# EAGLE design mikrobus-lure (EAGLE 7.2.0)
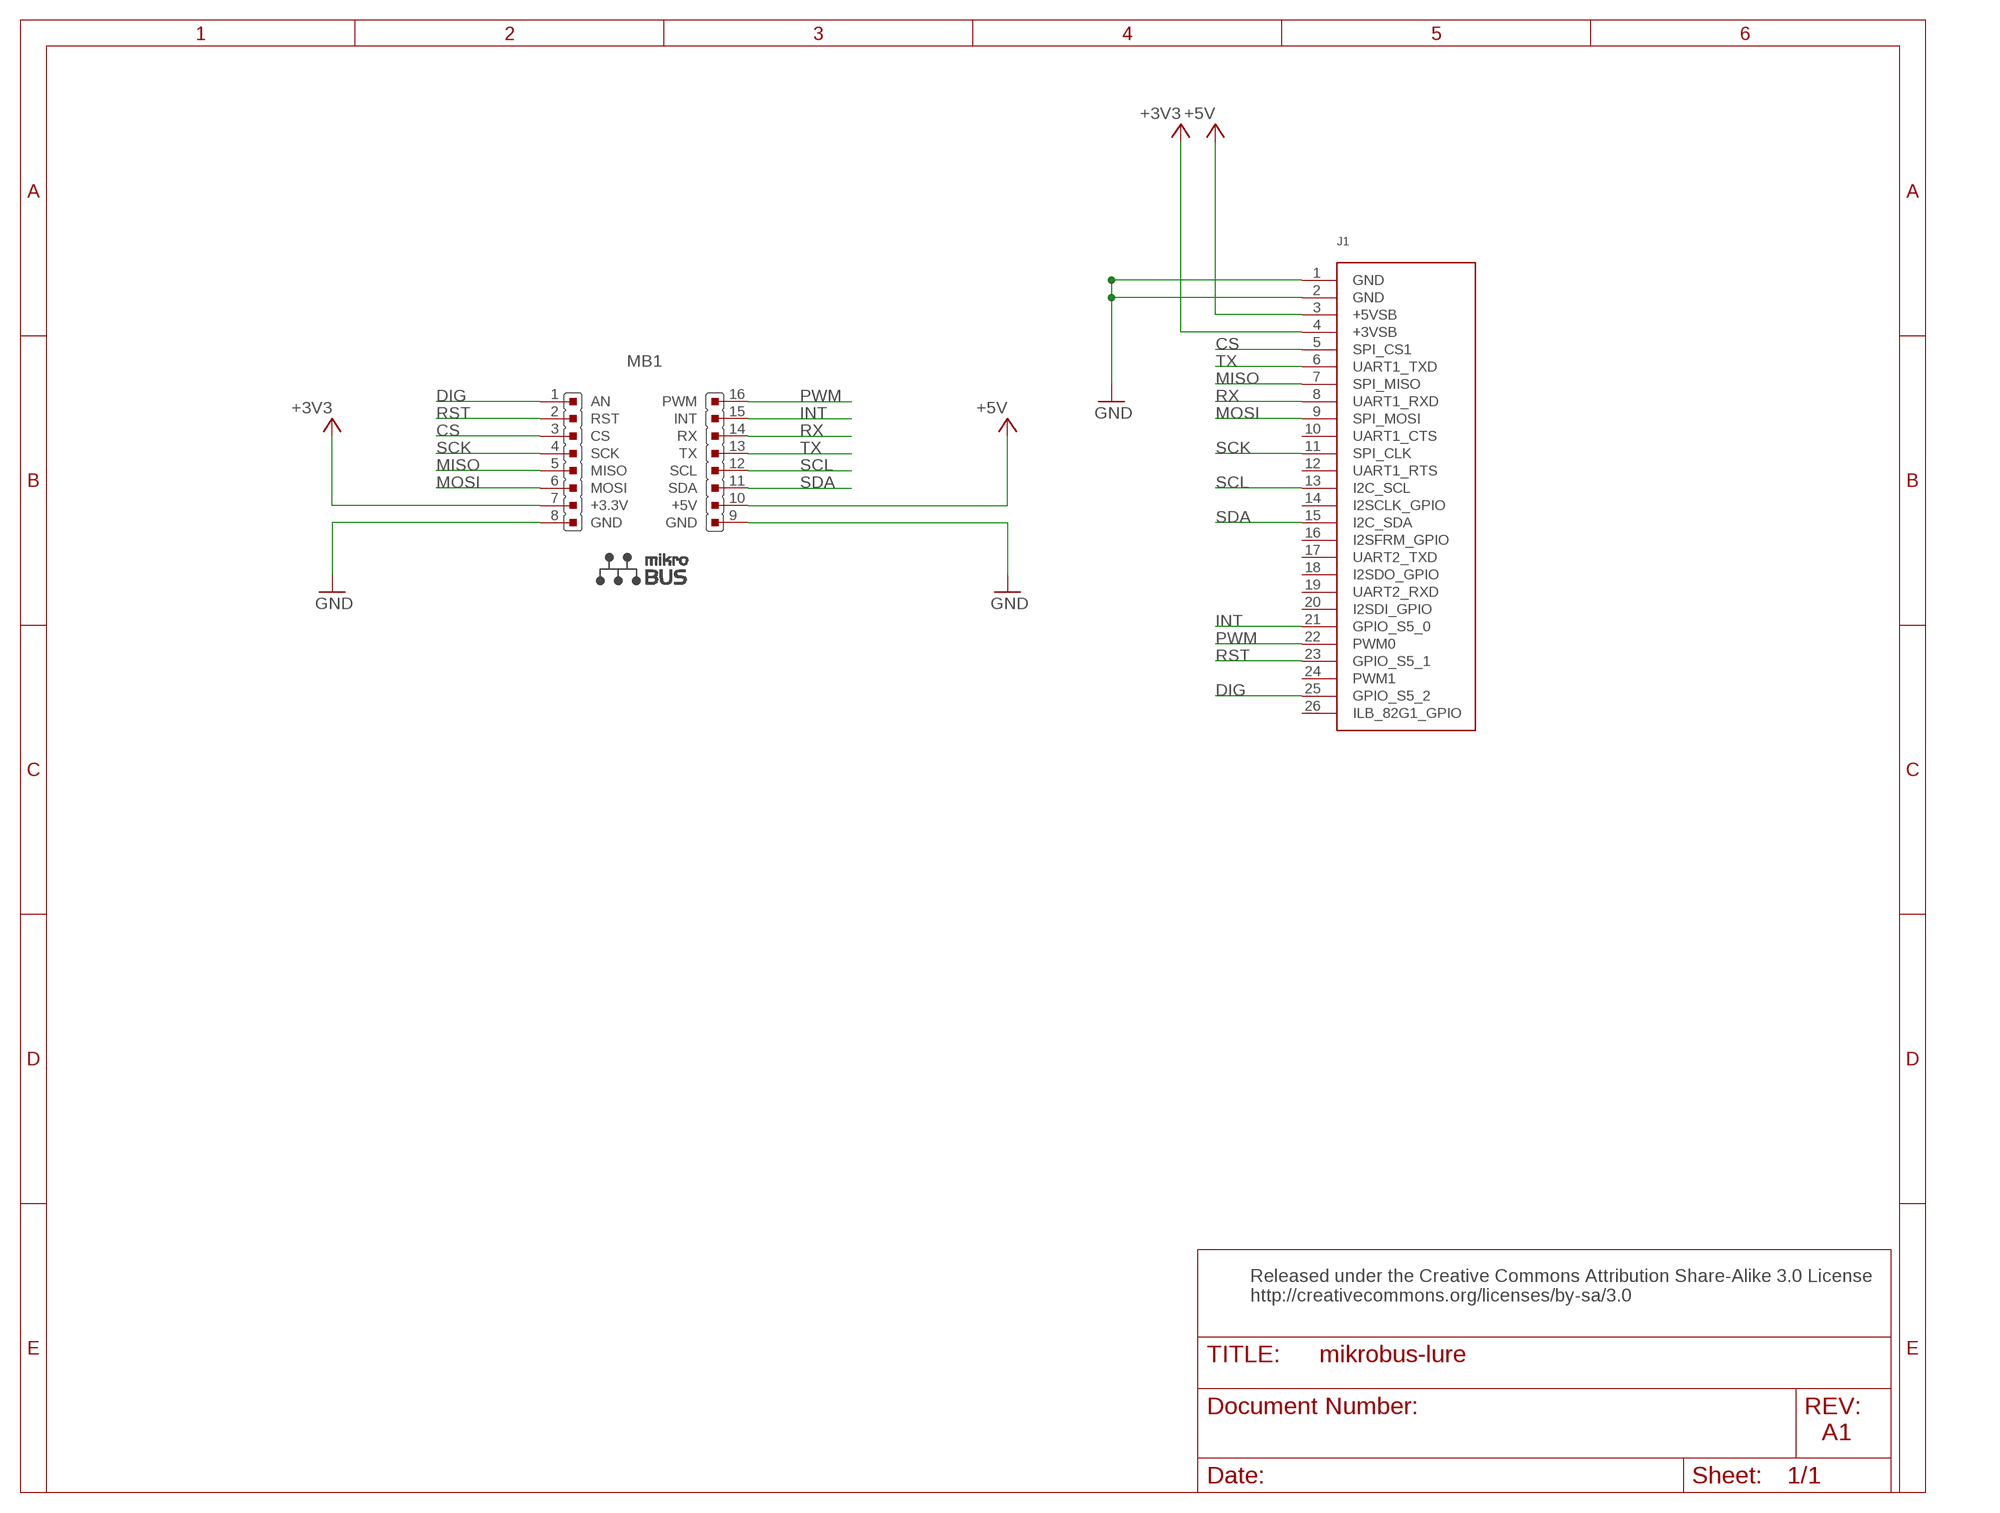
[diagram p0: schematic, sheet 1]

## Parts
J1  MBM_LSE  [MBM_LSE]
MB1  MIKROBUS  [MIKROBUS]

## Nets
+3V3: J1.4(+3VSB) MB1.7(+3.3V)
+5V: J1.3(+5VSB) MB1.10(+5V)
CS: J1.5(SPI_CS1) MB1.3(CS)
DIG: J1.25(GPIO_S5_2) MB1.1(AN)
GND: J1.1(GND) J1.2(GND) MB1.8(GND) MB1.9(GND)
INT: J1.21(GPIO_S5_0) MB1.15(INT)
MISO: J1.7(SPI_MISO) MB1.5(MISO)
MOSI: J1.9(SPI_MOSI) MB1.6(MOSI)
PWM: J1.22(PWM0) MB1.16(PWM)
RST: J1.23(GPIO_S5_1) MB1.2(RST)
RX: J1.8(UART1_RXD) MB1.14(RX)
SCK: J1.11(SPI_CLK) MB1.4(SCK)
SCL: J1.13(I2C_SCL) MB1.12(SCL)
SDA: J1.15(I2C_SDA) MB1.11(SDA)
TX: J1.6(UART1_TXD) MB1.13(TX)
Unconnected: J1.10(UART1_CTS) J1.12(UART1_RTS) J1.14(I2SCLK_GPIO) J1.16(I2SFRM_GPIO) J1.17(UART2_TXD) J1.18(I2SDO_GPIO) J1.19(UART2_RXD) J1.20(I2SDI_GPIO) J1.24(PWM1) J1.26(ILB_82G1_GPIO)

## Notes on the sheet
- Released under the Creative Commons Attribution Share-Alike 3.0 License
  http://creativecommons.org/licenses/by-sa/3.0
- A1

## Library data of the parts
J1 = mini-lse-lure:MBM_LSE
MB1 = MikroBUS:MIKROBUS: MikroBUS Source: MikroBUS specification MikroBUS

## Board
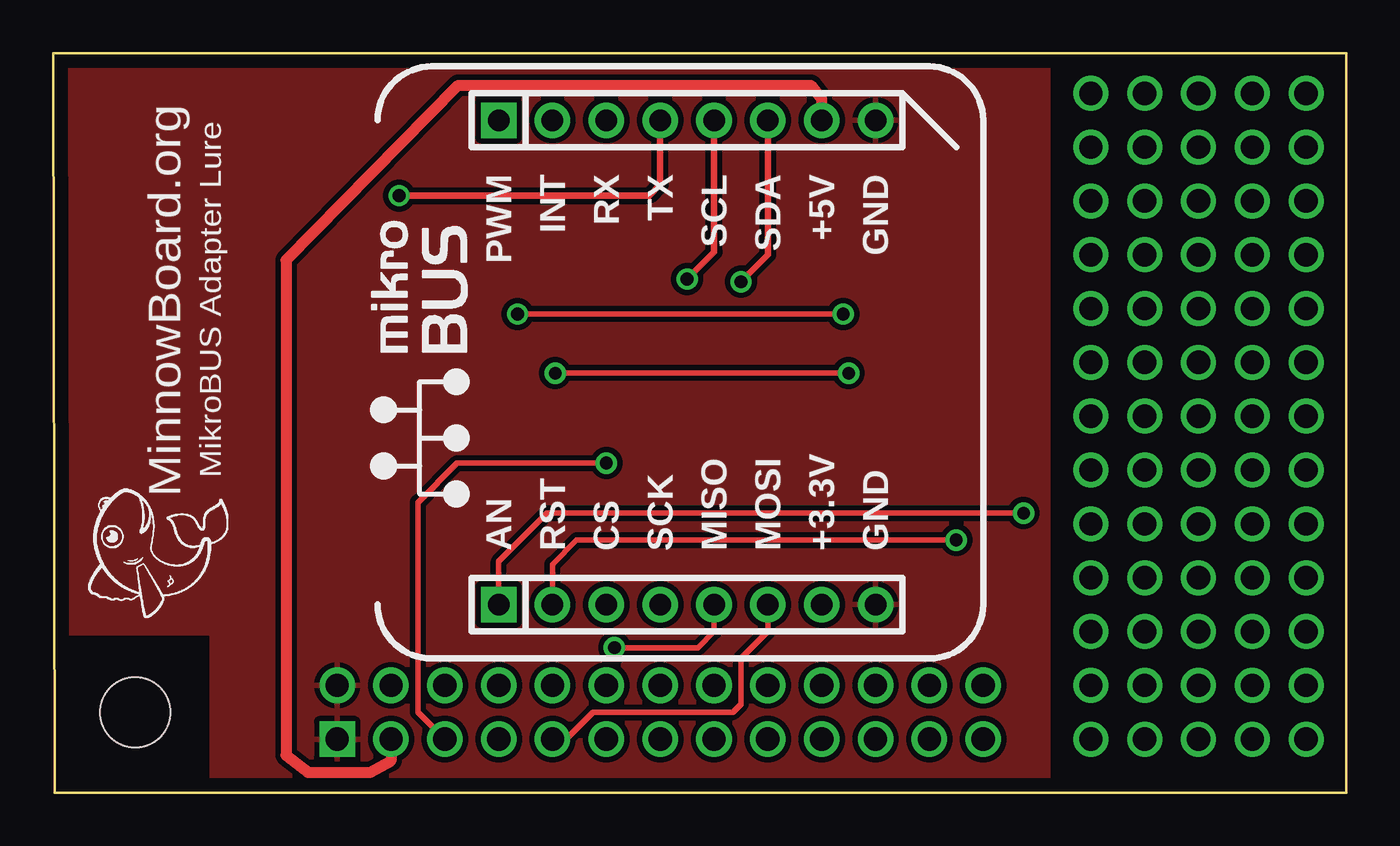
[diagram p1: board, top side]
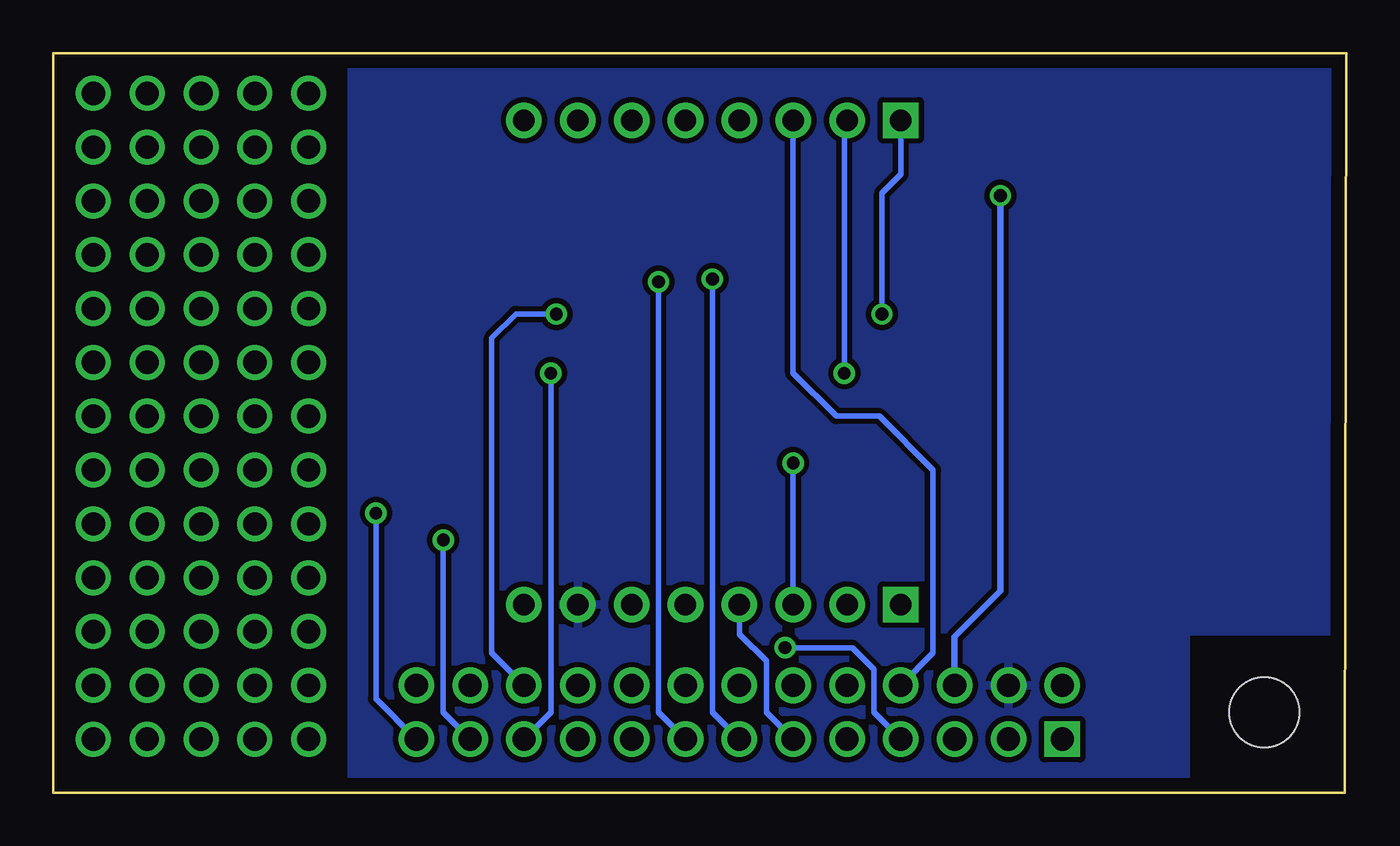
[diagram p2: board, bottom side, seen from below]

Size 61.04 x 34.92 mm. Coordinates in mm from the lower left corner, seen from the top.
Copper layers (1*16): Top 0.035mm / dielectric 1.5mm / Bottom 0.035mm
Design rules "default *": minimum track width 10mil, minimum drill 24mil, track to track 10mil, track to pad 10mil, pad to pad 10mil, via to via 10mil, smd to smd 8mil, copper to edge 25mil, drill to drill 8mil, minimum pad ring 0mil, minimum via ring 8mil, stop-mask expansion 4mil, vias tented up to drill 0mil, thermal gap 10mil

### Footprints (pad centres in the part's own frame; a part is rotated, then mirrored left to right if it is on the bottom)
MBM_LSE = drill 1.1 pad 1.676 square: 1 -15.24,0 | drill 1.1 pad 1.676: 2 -15.24,2.54; 3 -12.7,0; 4 -12.7,2.54; 5 -10.16,0; 6 -10.16,2.54; 7 -7.62,0; 8 -7.62,2.54; 9 -5.08,0; 10 -5.08,2.54; 11 -2.54,0; 12 -2.54,2.54; 13 0,0; 14 0,2.54; 15 2.54,0; 16 2.54,2.54; 17 5.08,0; 18 5.08,2.54; 19 7.62,0; 20 7.62,2.54; 21 10.16,0; 22 10.16,2.54; 23 12.7,0; 24 12.7,2.54; 25 15.24,0; 26 15.24,2.54 | hole 3.302: -24.765,1.27
MIKROBUS = drill 1.016 pad 1.676 square: 1 -11.43,7.62; 16 11.43,7.62 | drill 1.016 pad 1.676: 2 -11.43,5.08; 3 -11.43,2.54; 4 -11.43,0; 5 -11.43,-2.54; 6 -11.43,-5.08; 7 -11.43,-7.62; 8 -11.43,-10.16; 9 11.43,-10.16; 10 11.43,-7.62; 11 11.43,-5.08; 12 11.43,-2.54; 13 11.43,0; 14 11.43,2.54; 15 11.43,5.08

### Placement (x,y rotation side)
J1  28.65,2.54 0 top
MB1  28.65,20.32 90 top
U$1  [MINNOWBOARD_LOGO]  8.25,7.95 90 top

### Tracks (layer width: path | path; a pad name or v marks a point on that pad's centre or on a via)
+3V3
  pour Bottom: 0.08,34.92 46.94,34.92 46.94,0 0.08,0
+5V
  Top 0.508: J1.3 15.95,1.52 14.96,0.96 12.04,0.96 11,1.78 11,25.15 19.13,33.4 35.76,33.4 36.27,32.77 MB1.10
CS  (via drill 0.6)
  Top 0.254: J1.5 17.22,3.81 17.22,13.72 19.08,15.57 v26.11,15.57
  Bottom 0.254: v26.11,15.57 MB1.3
DIG  (via drill 0.6)
  Top 0.254: MB1.1 21.03,10.92 23.32,13.21 v45.8,13.21
  Bottom 0.254: v45.8,13.21 45.8,4.45 J1.25
GND
  pour Top: 0.08,34.92 46.94,34.92 46.94,0 0.08,0
INT  (via drill 0.6)
  Top 0.254: v37.54,19.81 v23.7,19.81
  Bottom 0.254: J1.21 37.54,3.81 v37.54,19.81 | v23.7,19.81 23.7,31.75 MB1.15
MISO  (via drill 0.6)
  Top 0.254: v26.49,6.86 30.43,6.86 31.19,7.62 MB1.5
  Bottom 0.254: J1.7 22.3,3.81 22.3,5.84 23.32,6.86 v26.49,6.86
MOSI
  Top 0.254: J1.9 24.21,2.54 25.48,3.81 32.08,3.81 32.46,4.19 32.46,6.35 33.73,7.62 MB1.6
N$16  (via drill 1.1)
  other vias: 59.13,2.54
N$17  (via drill 1.1)
  other vias: 59.13,5.08
N$18  (via drill 1.1)
  other vias: 59.13,7.62
N$19  (via drill 1.1)
  other vias: 59.13,10.16
N$20  (via drill 1.1)
  other vias: 59.13,12.7
N$21  (via drill 1.1)
  other vias: 59.13,15.24
N$22  (via drill 1.1)
  other vias: 59.13,17.78
N$23  (via drill 1.1)
  other vias: 59.13,20.32
N$24  (via drill 1.1)
  other vias: 59.13,22.86
N$25  (via drill 1.1)
  other vias: 59.13,25.4
N$26  (via drill 1.1)
  other vias: 59.13,27.94
N$27  (via drill 1.1)
  other vias: 59.13,30.48
N$28  (via drill 1.1)
  other vias: 59.13,33.02
N$31  (via drill 1.1)
  other vias: 56.59,2.54
N$32  (via drill 1.1)
  other vias: 56.59,5.08
N$33  (via drill 1.1)
  other vias: 56.59,7.62
N$34  (via drill 1.1)
  other vias: 56.59,10.16
N$35  (via drill 1.1)
  other vias: 56.59,12.7
N$36  (via drill 1.1)
  other vias: 56.59,15.24
N$37  (via drill 1.1)
  other vias: 56.59,17.78
N$38  (via drill 1.1)
  other vias: 56.59,20.32
N$39  (via drill 1.1)
  other vias: 56.59,22.86
N$40  (via drill 1.1)
  other vias: 56.59,25.4
N$41  (via drill 1.1)
  other vias: 56.59,27.94
N$42  (via drill 1.1)
  other vias: 56.59,30.48
N$43  (via drill 1.1)
  other vias: 56.59,33.02
N$46  (via drill 1.1)
  other vias: 54.05,2.54
N$47  (via drill 1.1)
  other vias: 54.05,5.08
N$48  (via drill 1.1)
  other vias: 54.05,7.62
N$49  (via drill 1.1)
  other vias: 54.05,10.16
N$50  (via drill 1.1)
  other vias: 54.05,12.7
N$51  (via drill 1.1)
  other vias: 54.05,15.24
N$52  (via drill 1.1)
  other vias: 54.05,17.78
N$53  (via drill 1.1)
  other vias: 54.05,20.32
N$54  (via drill 1.1)
  other vias: 54.05,22.86
N$55  (via drill 1.1)
  other vias: 54.05,25.4
N$56  (via drill 1.1)
  other vias: 54.05,27.94
N$57  (via drill 1.1)
  other vias: 54.05,30.48
N$58  (via drill 1.1)
  other vias: 54.05,33.02
N$61  (via drill 1.1)
  other vias: 51.51,2.54
N$62  (via drill 1.1)
  other vias: 51.51,5.08
N$63  (via drill 1.1)
  other vias: 51.51,7.62
N$64  (via drill 1.1)
  other vias: 51.51,10.16
N$65  (via drill 1.1)
  other vias: 51.51,12.7
N$66  (via drill 1.1)
  other vias: 51.51,15.24
N$67  (via drill 1.1)
  other vias: 51.51,17.78
N$68  (via drill 1.1)
  other vias: 51.51,20.32
N$69  (via drill 1.1)
  other vias: 51.51,22.86
N$70  (via drill 1.1)
  other vias: 51.51,25.4
N$71  (via drill 1.1)
  other vias: 51.51,27.94
N$72  (via drill 1.1)
  other vias: 51.51,30.48
N$73  (via drill 1.1)
  other vias: 51.51,33.02
N$76  (via drill 1.1)
  other vias: 48.97,2.54
N$77  (via drill 1.1)
  other vias: 48.97,5.08
N$78  (via drill 1.1)
  other vias: 48.97,7.62
N$79  (via drill 1.1)
  other vias: 48.97,10.16
N$80  (via drill 1.1)
  other vias: 48.97,12.7
N$81  (via drill 1.1)
  other vias: 48.97,15.24
N$82  (via drill 1.1)
  other vias: 48.97,17.78
N$83  (via drill 1.1)
  other vias: 48.97,20.32
N$84  (via drill 1.1)
  other vias: 48.97,22.86
N$85  (via drill 1.1)
  other vias: 48.97,25.4
N$86  (via drill 1.1)
  other vias: 48.97,27.94
N$87  (via drill 1.1)
  other vias: 48.97,30.48
N$88  (via drill 1.1)
  other vias: 48.97,33.02
PWM  (via drill 0.6)
  Top 0.254: v37.29,22.61 v21.92,22.61
  Bottom 0.254: v21.92,22.61 21.92,28.32 21.03,29.21 MB1.16 | J1.22 40.34,6.6 40.34,21.46 39.19,22.61 v37.29,22.61
RST  (via drill 0.6)
  Top 0.254: MB1.2 23.57,10.79 24.71,11.94 v42.62,11.94
  Bottom 0.254: v42.62,11.94 42.62,3.81 J1.23
RX
  Bottom 0.254: J1.8 19.51,6.6 19.51,15.24 22.05,17.78 24.08,17.78 26.11,19.81 MB1.14
SCK
  Bottom 0.254: J1.11 27.38,3.81 27.38,6.22 28.65,7.49 MB1.4
SCL  (via drill 0.6)
  Top 0.305: v29.92,24.26 31.19,25.53 MB1.12
  Bottom 0.254: J1.13 29.92,3.81 v29.92,24.26
SDA  (via drill 0.6)
  Top 0.305: v32.46,24.13 33.73,25.4 MB1.11
  Bottom 0.254: J1.15 32.46,3.81 v32.46,24.13
TX  (via drill 0.6)
  Top 0.305: v16.33,28.19 28.14,28.19 28.65,28.7 MB1.13
  Bottom 0.305: J1.6 18.49,7.37 16.33,9.53 v16.33,28.19

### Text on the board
tPlace: MikroBUS Adapter Lure | MinnowBoard.org
Notes: Released under the Creative Commons Attribution Share-Alike 3.0 License / http://creativecommons.org/licenses/by-sa/3.0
